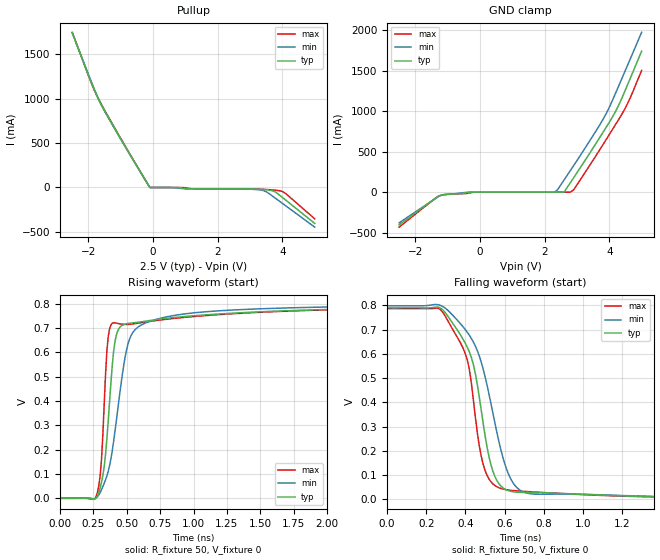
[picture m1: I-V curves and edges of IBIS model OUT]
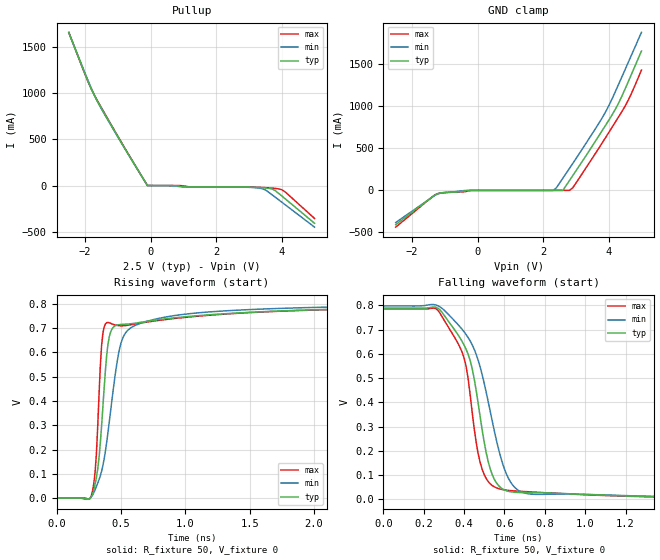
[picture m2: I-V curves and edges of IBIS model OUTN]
|   IBIS File of SG2016HHN D
|   HCSL Zdiff=100, Vcc=2.5V, fo>212.5MHz
[IBIS Ver]   3.2
[File Name]   sg2016hhn_hf_25v.ibs
[File Rev]   1.0
[Date]   Aug. 4, 2020
[Source]
[Notes]
Created by Minoru Kozaki
[Disclaimer]
Seiko Epson Corporation makes no warranty with respect to the
information contained herein.
[Copyright]
Copyright(C) 2020, Seiko Epson Corporation. All rights reserved.
|   Component
[Component]   SG2016HHN
[Manufacturer]  Seiko Epson Corporation
[Package]
R_pkg   8.9m   NA   NA
L_pkg   197p   NA   NA
C_pkg   267f   NA   NA
[Pin]   signal_name   model_name   R_pin   L_pin   C_pin
1   OE/ST   NC
2   NC   NC
3   GND   GND
4   OUT   OUT   8.9m   197p   267f
5   OUTN   OUTN   9.9m   222p   245f
6   VCC   POWER
[Diff Pin] inv_pin  vdiff  tdelay_typ
4   5   0   0
| Models and submodels in the file (2): OUT (Open_source), OUTN (Open_source)
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|   Model OUT
[Model]   OUT
Model_type   Open_source
Polarity   Non-Inverting
Vref = 0
Vmeas = 0.4
Rref = 50
Cref = 0
C_comp   12.0p   12.0p   12.0p
[Temperature Range]   25   105   -40
[Voltage Range]   2.5   2.25   2.75
[Pullup Reference]   2.5   2.25   2.75
[GND Clamp Reference]   0   0   0
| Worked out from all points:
|   GND clamp passes 1 mA (typ) near -0.25 V on its own axis
|   falling waveform, R_fixture 50, V_fixture 0: 20-80 % time 119ps typ, 149ps min, 102ps max; typ from 0.79 V to 0 V
|   rising waveform, R_fixture 50, V_fixture 0: 20-80 % time 71.7ps typ, 131ps min, 44.6ps max; typ from 0 V to 0.788 V
[Pullup]
-2.5V     1.739A     1.738A     1.746A
-1.9V     1.169A     1.18A      1.166A
-1.7V     1A         1.006A     1.004A
-1.5V     861.7mA    859.3mA    870.7mA
-1.3V     734.6mA    730.6mA    742.6mA
-100mV    31.31uA    15.33uA    89.14uA
1V        -12.37mA   -15.31mA   -2.908mA
2.9V      -16.64mA   -17.92mA   -16.19mA
3.4V      -22.68mA   -33.6mA    -20.86mA
3.7V      -37.07mA   -98.63mA   -27.47mA
4V        -112.1mA   -178.6mA   -45mA
5V        -404.4mA   -446.2mA   -352.5mA
[GND Clamp]
-2.5V     -403.1mA   -378.3mA   -431.7mA
-1.2V     -36.21mA   -38.92mA   -37.68mA
-300mV    -1.759mA   -603.5uA   -8.211mA
2.3V      -1.475uA   3.582uA    -3.007uA
2.4V      -1.333uA   29.72mA    -2.745uA
2.6V      31.31uA    149mA      -2.258uA
2.8V      119.4mA    268.7mA    13.29uA
2.9V      179.5mA    328.8mA    29.86mA
3.8V      734.6mA    893.4mA    583.2mA
4.2V      1A         1.226A     838.6mA
4.6V      1.358A     1.598A     1.122A
5V        1.739A     1.971A     1.502A
[Falling Waveform]
R_fixture = 50
V_fixture = 0
V_fixture_min = 0
V_fixture_max = 0
0s        789.6mV    798.5mV    786.6mV
270ps     790.2mV    800.8mV    784.1mV
410ps     626.2mV    688.3mV    572.6mV
450ps     520.4mV    633.1mV    341.7mV
470ps     424.5mV    592.3mV    222.5mV
500ps     262.8mV    506.2mV    118.9mV
550ps     94.37mV    315.4mV    57.15mV
630ps     33.46mV    85.7mV     37.57mV
760ps     27.93mV    21.44mV    30.1mV
4ns       291uV      396uV      253uV
[Rising Waveform]
R_fixture = 50
V_fixture = 0
V_fixture_min = 0
V_fixture_max = 0
0s        115uV      153uV      111uV
280ps     9.556mV    6.81mV     24.77mV
310ps     65.91mV    35.5mV     159.1mV
340ps     178.9mV    75.59mV    506mV
360ps     314.8mV    109.9mV    662.8mV
400ps     600.2mV    230.8mV    722.1mV
440ps     697.3mV    401mV      718.4mV
520ps     720mV      654.3mV    715.6mV
710ps     734.1mV    734.4mV    730.4mV
4ns       788.4mV    797.1mV    785.7mV
[Ramp]
R_load = 50
dV/dt_r   0.47612/71.83p   0.48039/131.82p   0.47496/43.85p
dV/dt_f   0.47612/119.99p   0.48039/149.77p   0.47496/101.63p
|   Model OUTN
[Model]   OUTN
Model_type   Open_source
Polarity   Inverting
Vref = 0
Vmeas = 0.4
Rref = 50
Cref = 0
C_comp   12.0p   12.0p   12.0p
[Temperature Range]   25   105   -40
[Voltage Range]   2.5   2.25   2.75
[Pullup Reference]   2.5   2.25   2.75
[GND Clamp Reference]   0   0   0
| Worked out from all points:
|   GND clamp passes 1 mA (typ) near -0.25 V on its own axis
|   falling waveform, R_fixture 50, V_fixture 0: 20-80 % time 116ps typ, 147ps min, 99.6ps max; typ from 0.789 V to 0 V
|   rising waveform, R_fixture 50, V_fixture 0: 20-80 % time 70.8ps typ, 131ps min, 43.8ps max; typ from 0 V to 0.788 V
[Pullup]
-2.5V     1.655A     1.655A     1.659A
-2V       1.203A     1.213A     1.2A
-1.7V     960.9mA    964.5mA    966.4mA
-1.2V     648.2mA    644.8mA    654.9mA
-100mV    31.32uA    15.33uA    89.15uA
1V        -12.33mA   -15.3mA    -2.901mA
1.2V      -15.35mA   -15.77mA   -14.67mA
2.9V      -16.63mA   -17.91mA   -16.19mA
3.4V      -22.68mA   -33.59mA   -20.86mA
3.7V      -37.08mA   -99.23mA   -27.48mA
4V        -113mA     -180.1mA   -45.08mA
5V        -408.6mA   -450.4mA   -356.6mA
[GND Clamp]
-2.5V     -407.4mA   -381.8mA   -436.7mA
-1.2V     -36.22mA   -38.92mA   -37.71mA
-300mV    -1.757mA   -603.2uA   -8.165mA
2.3V      -1.475uA   3.582uA    -3.007uA
2.4V      -1.333uA   28.69mA    -2.745uA
2.6V      31.32uA    143.8mA    -2.258uA
2.8V      115.3mA    259.4mA    13.29uA
2.9V      173.3mA    317.4mA    28.82mA
3.9V      769.9mA    928.2mA    624.1mA
4.2V      960.9mA    1.169A     809.2mA
4.5V      1.203A     1.434A     1A
5V        1.655A     1.877A     1.429A
[Falling Waveform]
R_fixture = 50
V_fixture = 0
V_fixture_min = 0
V_fixture_max = 0
0s        789mV      797.8mV    786mV
260ps     792.4mV    801.8mV    786.5mV
370ps     678.6mV    720.8mV    643mV
410ps     618.8mV    679.7mV    548.6mV
460ps     448.5mV    598mV      234.1mV
490ps     284.2mV    512.8mV    122.7mV
540ps     100.9mV    320.9mV    56.95mV
620ps     33.19mV    86.56mV    37.05mV
750ps     27.65mV    20.89mV    29.95mV
4ns       285uV      386uV      249uV
[Rising Waveform]
R_fixture = 50
V_fixture = 0
V_fixture_min = 0
V_fixture_max = 0
0s        110uV      157uV      109uV
270ps     4.659mV    5.235mV    8.758mV
290ps     35.57mV    22.6mV     61.76mV
310ps     85.74mV    47.89mV    185.3mV
350ps     297mV      110.5mV    627.4mV
390ps     589.4mV    231.3mV    721.6mV
430ps     694.7mV    401.8mV    716.5mV
500ps     714.2mV    636.2mV    708.7mV
690ps     726mV      725.1mV    722.9mV
4ns       787.7mV    796.3mV    785.1mV
[Ramp]
R_load = 50
dV/dt_r   0.47608/71.41p   0.48035/132.84p   0.47490/43.85p
dV/dt_f   0.47608/117.79p   0.48035/147.92p   0.47490/101.63p
